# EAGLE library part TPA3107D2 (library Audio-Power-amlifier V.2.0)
15-W STEREO CLASS-D AUDIO POWER AMPLIFIER
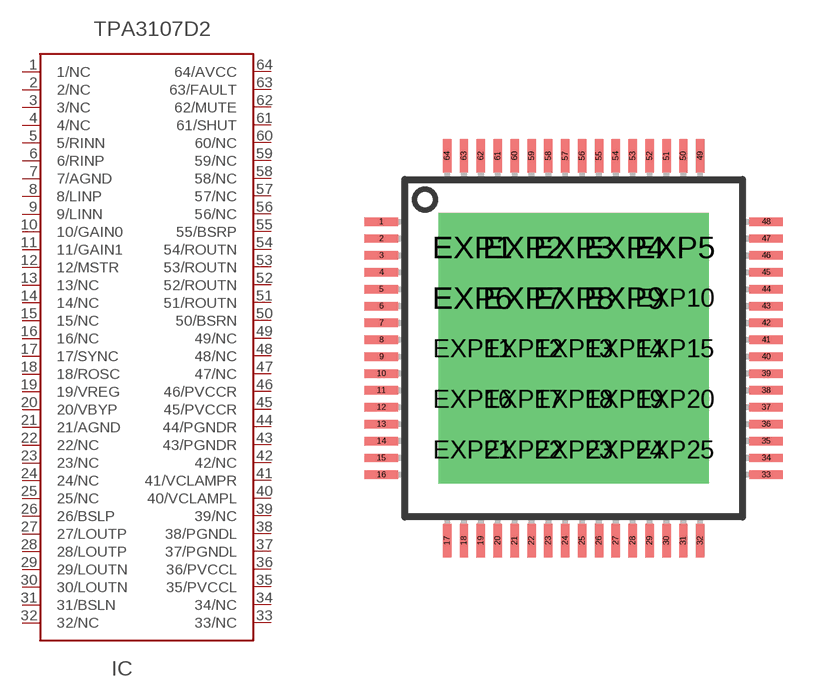
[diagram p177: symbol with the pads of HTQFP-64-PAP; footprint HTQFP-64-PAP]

Designator prefix IC

## TPA3107D2  [HTQFP-64-PAP]
1  1/NC  nc
2  2/NC  nc
3  3/NC  nc
4  4/NC  nc
5  5/RINN  in
6  6/RINP  in
7  7/AGND  pwr
8  8/LINP  in
9  9/LINN  in
10  10/GAIN0  in
11  11/GAIN1  in
12  12/MSTR  in
13  13/NC  nc
14  14/NC  nc
15  15/NC  nc
16  16/NC  nc
17  17/SYNC
18  18/ROSC
19  19/VREG  out
20  20/VBYP  out
21  21/AGND  pwr
22  22/NC  nc
23  23/NC  nc
24  24/NC  nc
25  25/NC  nc
26  26/BSLP
27  27/LOUTP  out
28  28/LOUTP  out
29  29/LOUTN  out
30  30/LOUTN  out
31  31/BSLN
32  32/NC  nc
33  33/NC  nc
34  34/NC  nc
35  35/PVCCL  pwr
36  36/PVCCL  pwr
37  37/PGNDL  pwr
38  38/PGNDL  pwr
39  39/NC  nc
40  40/VCLAMPL  pwr
41  41/VCLAMPR  pwr
42  42/NC  nc
43  43/PGNDR  pwr
44  44/PGNDR  pwr
45  45/PVCCR  pwr
46  46/PVCCR  pwr
47  47/NC  nc
48  48/NC  nc
49  49/NC  nc
50  50/BSRN
51  51/ROUTN  out
52  52/ROUTN  out
53  53/ROUTN  out
54  54/ROUTN  out
55  55/BSRP
56  56/NC  nc
57  57/NC  nc
58  58/NC  nc
59  59/NC  nc
60  60/NC  nc
61  61/SHUT  in
62  62/MUTE  in
63  63/FAULT  out
64  64/AVCC  pwr

## Footprint HTQFP-64-PAP (pad centres in mm)
PAP (S-PQFP-G46) PowerPAD Package Source: http://focus.ti.com/lit/ds/symlink/ads1274.pdf www.ti.com .. slma002.pdf
smd 1 x 0.25: 1 -5.7,3.75; 2 -5.7,3.25; 3 -5.7,2.75; 4 -5.7,2.25; 5 -5.7,1.75; 6 -5.7,1.25; 7 -5.7,0.75; 8 -5.7,0.25; 9 -5.7,-0.25; 10 -5.7,-0.75; 11 -5.7,-1.25; 12 -5.7,-1.75; 13 -5.7,-2.25; 14 -5.7,-2.75; 15 -5.7,-3.25; 16 -5.7,-3.75; 33 5.7,-3.75; 34 5.7,-3.25; 35 5.7,-2.75; 36 5.7,-2.25; 37 5.7,-1.75; 38 5.7,-1.25; 39 5.7,-0.75; 40 5.7,-0.25; 41 5.7,0.25; 42 5.7,0.75; 43 5.7,1.25; 44 5.7,1.75; 45 5.7,2.25; 46 5.7,2.75; 47 5.7,3.25; 48 5.7,3.75
smd 0.25 x 1: 17 -3.75,-5.7; 18 -3.25,-5.7; 19 -2.75,-5.7; 20 -2.25,-5.7; 21 -1.75,-5.7; 22 -1.25,-5.7; 23 -0.75,-5.7; 24 -0.25,-5.7; 25 0.25,-5.7; 26 0.75,-5.7; 27 1.25,-5.7; 28 1.75,-5.7; 29 2.25,-5.7; 30 2.75,-5.7; 31 3.25,-5.7; 32 3.75,-5.7; 49 3.75,5.7; 50 3.25,5.7; 51 2.75,5.7; 52 2.25,5.7; 53 1.75,5.7; 54 1.25,5.7; 55 0.75,5.7; 56 0.25,5.7; 57 -0.25,5.7; 58 -0.75,5.7; 59 -1.25,5.7; 60 -1.75,5.7; 61 -2.25,5.7; 62 -2.75,5.7; 63 -3.25,5.7; 64 -3.75,5.7
drill 0.3 pad 2 square: EXP1 -3,3; EXP2 -1.5,3; EXP3 0,3; EXP4 1.5,3; EXP5 3,3; EXP6 -3,1.5; EXP7 -1.5,1.5; EXP8 0,1.5; EXP9 1.5,1.5; EXP10 3,1.5; EXP11 -3,0; EXP12 -1.5,0; EXP13 0,0; EXP14 1.5,0; EXP15 3,0; EXP16 -3,-1.5; EXP17 -1.5,-1.5; EXP18 0,-1.5; EXP19 1.5,-1.5; EXP20 3,-1.5; EXP21 -3,-3; EXP22 -1.5,-3; EXP23 0,-3; EXP24 1.5,-3; EXP25 3,-3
